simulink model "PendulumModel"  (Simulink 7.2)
settings: Solver=ode3  StartTime=0.0  StopTime=100  FixedStep=0.1  RelTol=1e-3
PreLoadFcn:
  | pid=readfis('pid.fis');
undefined symbols (not defined in the file or in its folder): deg, kg, m, s
libraries: mblibv1 x6

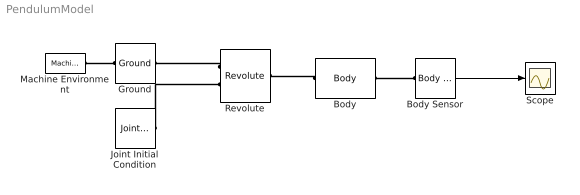
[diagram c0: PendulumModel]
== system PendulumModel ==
  Body : mblibv1/Bodies/Body  DialogController=MECH.DynMechDlgSource  PhysicalDomain=mechanical  SubClassName=Unknown  LeftPortType=workingframe  RightPortType=workingframe  LConnTagsString=CS1  RConnTagsString=CS2  UpdateFromCAD=off  DialogClass=MechanicalBodyBlock  Mass=1  MassUnits=kg  InertiaUnits=kg*m^2  Inertia=eye(3)  Shape=Cylinder  ShapeDims=[1 1]  ShapeUnits=m  ShapeUse=false  Density=1  DensityUnits=kg/m^3  DensityUse=false  GraphicsMode=MACHINE_DEFAULT  BodyColorSelMode=MACHINE_DEFAULT  BodyColor=[1 0 0]  AttachedToCS=CG  CG=Left$CG$[0 -1 0]$WORLD$WORLD$m$[0 0 0]$Euler X-Y-Z$deg$WORLD$false$none  WorkingFrames=Left$CS1$[0 0 0]$World$World$m$[0 0 0]$Euler X-Y-Z$deg$WORLD$true$none#Right$CS2$[0 -2 0]$World$World$m$[0 0 0]$Euler X-Y-Z$deg$WORLD$true$none  CGPos=[0 -1 0]  CGRot=[0 0 0]  CS0Pos=[]  CS0Rot=[]  CS1Pos=[0 0 0]  CS1Rot=[0 0 0]  CS2Pos=[0 -2 0]  CS2Rot=[0 0 0]  CS3Pos=[]  CS3Rot=[]  CS4Pos=[]  CS4Rot=[]  CS5Pos=[]  CS5Rot=[]  CS6Pos=[]  CS6Rot=[]  CS7Pos=[]  CS7Rot=[]  CS8Pos=[]  CS8Rot=[]  CS9Pos=[]  CS9Rot=[]  CS10Pos=[]  CS10Rot=[]  CS11Pos=[]  CS11Rot=[]  CS12Pos=[]  CS12Rot=[]  CS13Pos=[]  CS13Rot=[]  CS14Pos=[]  CS14Rot=[]  CS15Pos=[]  CS15Rot=[]  CS16Pos=[]  CS16Rot=[]  CS17Pos=[]  CS17Rot=[]  CS18Pos=[]  CS18Rot=[]  CS19Pos=[]  CS19Rot=[]  CS20Pos=[]  CS20Rot=[]
  Body Sensor : mblibv1/Sensors &  Actuators/Body Sensor  DialogController=MECH.DynMechDlgSource  SystemSampleTime=-1  UpdateFromCAD=off  PhysicalDomain=Mechanical  PortType=blob  Muxed=on  Pose=off  Angle=on  AngleUnits=deg  ArcVelocity=off  ArcVelocityUnits=deg/s  ArcAcceleration=off  ArcAccelerationUnits=deg/s^2  CoordPosition=on  CoordPositionUnits=m  Velocity=off  VelocityUnits=m/s  Acceleration=off  AccelerationUnits=m/s^2  Quaternion=on  QuaternionDT=off  QuaternionDDT=off  QuaternionUnits=off  OutputVector=[1]  ActiveIO=on  Width=3  DialogClass=MechanicalSensorBlock  ReferenceFrame=Absolute (World)
  Ground : mblibv1/Bodies/Ground  DialogController=MECH.DynMechDlgSource  SystemSampleTime=-1  UpdateFromCAD=off  LeftPortType=env  RightPortType=workingframe  PhysicalDomain=Mechanical  DialogClass=GroundBlock  CoordPosition=[0 0 0]  CoordPositionUnits=m  StateVectorMgrId=0  MachineId=[1 0]  ShowEnvPort=on
  Joint Initial Condition : mblibv1/Sensors &  Actuators/Joint Initial Condition  DialogController=MECH.DynMechDlgSource  SystemSampleTime=-1  UpdateFromCAD=off  PhysicalDomain=mechanical  DialogClass=InitialConditionBlock  InitialConditions=P1$false$0$m$deg$0$m/s$deg/s#P2$false$0$m$deg$0$m/s$deg/s#P3$false$0$m$deg$0$m/s$deg/s#R1$true$10$m$deg$0$m/s$deg/s#R2$false$0$m$deg$0$m/s$deg/s#R3$false$0$m$deg$0$m/s$deg/s#S$false$0$m$deg$0$m/s$deg/s  P1PIC=0  P1VIC=0  P2PIC=0  P2VIC=0  P3PIC=0  P3VIC=0  R1PIC=10  R1VIC=0  R2PIC=0  R2VIC=0  R3PIC=0  R3VIC=0  SPIC=0  SVIC=0
  Machine Environment : mblibv1/Bodies/Machine Environment  Tag=Factory ground  DialogController=MECH.DialogSource  SystemSampleTime=-1  PortType=env  PhysicalDomain=Mechanical  DialogTemplateClass=MECH.MachineEnvironment  SyncWhenCopied=off  Gravity=[0 -9.81 0]  GravityUnits=m/s^2  GravityAsSignal=off  Dimensionality=Auto-detect  AnalysisType=Forward dynamics  LinearAssemblyTolerance=1e-3  LinearAssemblyToleranceUnits=m  AngularAssemblyTolerance=1e-3  AngularAssemblyToleranceUnits=rad  ConstraintSolverType=Stabilizing  ConstraintRelTolerance=1e-4  ConstraintAbsTolerance=1e-4  UseRobustSingularityHandling=off  RedundancyAnalysisToleranceType=Automatically select tolerance  RedundancyAnalysisTolerance=1e-14  StatePerturbationType=Fixed  PerturbationSize=1e-5  VisualizeMachine=on  BodyVisualizationType=Use model default body geometries  BodyColorSelMode=Use model default  DefaultBodyColor=[1 0 0]
  Revolute : mblibv1/Joints/Revolute  DialogController=MECH.DynMechDlgSource  PhysicalDomain=mechanical  SubClassName=Unknown  LeftPortType=blob  RightPortType=blob  LConnTagsString=__newl0|SA1  RConnTagsString=__newr0  UpdateFromCAD=off  NumSAPorts=1  CutJoint=off  MarkAsCut=off  Primitives=prismatic  PrimitiveProps=R1$World$[0 0 1]$revolute  DialogClass=JointBlock  R1Axis=[0 0 1]
  Scope : Scope
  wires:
  Body Sensor/1 -> Scope/1
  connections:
  Machine Environment/RConn1 -- Ground/LConn1
  Revolute/LConn1 -- Ground/RConn1
  Body/LConn1 -- Revolute/RConn1
  Body Sensor/LConn1 -- Body/RConn1
  Joint Initial Condition/RConn1 -- Revolute/LConn2
